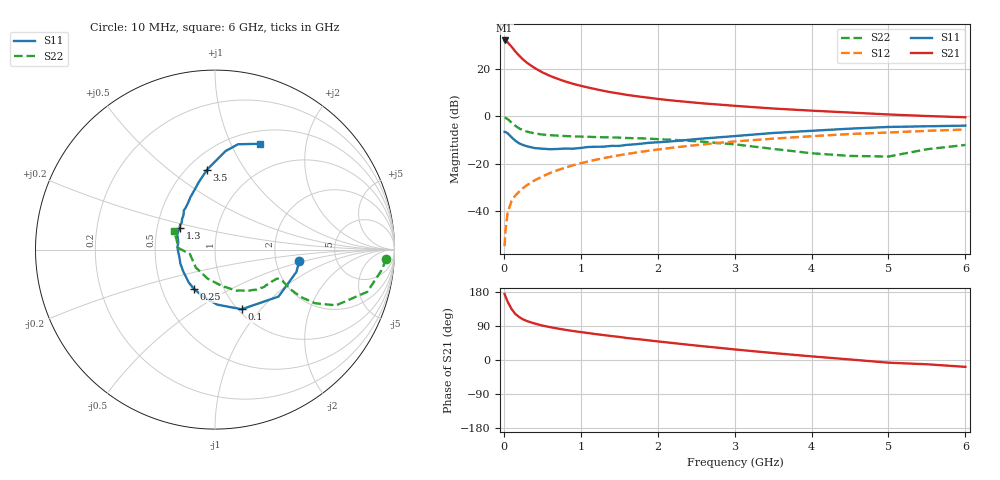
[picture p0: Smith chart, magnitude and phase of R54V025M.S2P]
! SIEMENS Small Signal Semiconductors
! BFR183
! Si NPN RF Bipolar Junction Transistor in SOT23
! VCE = 4 V  IC = 25 mA
! Common Emitter S-Parameters:  May  1996
# GHz  S  MA  R  50
!  f  S11  S21  S12  S22
! GHz  MAG  ANG  MAG  ANG  MAG  ANG  MAG  ANG
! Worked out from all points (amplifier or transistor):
!   36 points, 10 MHz to 6 GHz, reference 50 ohm
!   highest |S21| = 32.2 dB at 10 MHz (marker M1)
!   |S21| within 3 dB of that: start of sweep to 108.8 MHz
!   unconditionally stable (mu >= 1): 484.5 MHz to 2.371 GHz
!   at 250 MHz: K = 0.85, MSG = 27.2 dB, |S12| = -30.3 dB
!   at 1.4 GHz: K = 1.04, MAG = 12.3 dB, |S12| = -17.0 dB
!   at 6 GHz: K = 0.90, MSG = 2.6 dB, |S12| = -5.5 dB
!   S11 on the Smith chart (normalised r, x): 10 MHz: 2.71, -0.46; 100 MHz: 1.04, -0.80; 250 MHz: 0.72, -0.34; 1.3 GHz: 0.66, +0.17; 3.5 GHz: 0.62, +0.69; 6 GHz: 0.65, +1.30
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0.01  0.4737 -7.9  40.65 174.0  0.0018 87.4  0.954 -3.0
0.02  0.4705 -15.3  40.14 168.5  0.0037 81.6  0.9389 -6.6
0.05  0.4402 -36.5  37.16 153.6  0.0093 77.4  0.8804 -15.5
0.1  0.3641 -65.9  29.99 134.6  0.0162 72.9  0.743 -24.7
0.15  0.3067 -87.8  23.71 121.5  0.0213 69.7  0.6327 -28.2
0.2  0.2695 -104.4  19.34 113.2  0.0257 69.8  0.5598 -28.8
0.25  0.2486 -118.2  16.06 107.2  0.0305 70.2  0.5087 -28.4
0.3  0.2341 -128.8  13.74 102.8  0.0351 71.3  0.4777 -27.7
0.4  0.2144 -146.0  10.62 96.3  0.0445 72.1  0.4386 -26.1
0.5  0.208 -158.0  8.589 90.9  0.0536 73.3  0.4145 -24.9
0.6  0.2029 -167.8  7.241 86.8  0.0636 73.0  0.4017 -24.6
0.7  0.2053 -176.6  6.262 83.0  0.0733 72.7  0.3933 -24.7
0.8  0.2099 176.2  5.497 79.6  0.0828 71.9  0.385 -24.9
0.9  0.2081 169.3  4.914 76.5  0.0928 71.5  0.3795 -25.3
1.1  0.2262 158.8  4.086 71.0  0.1122 70.2  0.3714 -27.4
1.3  0.2297 148.7  3.478 65.7  0.1318 68.5  0.3629 -29.4
1.7  0.2571 133.6  2.717 55.8  0.1703 64.6  0.3467 -35.0
2.2  0.2995 120.2  2.169 44.7  0.2191 58.9  0.3214 -43.9
3.5  0.4474 95.7  1.475 18.4  0.3391 42.4  0.2061 -79.3
4.5  0.5528 83.8  1.212 1.4  0.4259 29.7  0.1463 -136.7
5.5  0.6201 71.6  1.023 -11.3  0.4968 18.0  0.2025 177.7
6  0.6407 66.9  0.962 -18.1  0.5303 10.5  0.2499 155.3
